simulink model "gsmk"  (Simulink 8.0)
settings: Solver=ode45  SolverMode=SingleTasking  StartTime=0.0  StopTime=3.0  RelTol=1e-3  AbsTol=1e-6
undefined symbols (not defined in the file or in its folder): DiscIntNeverNeededParam

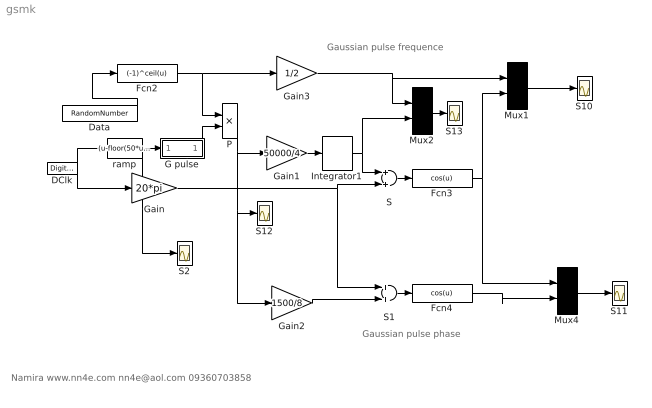
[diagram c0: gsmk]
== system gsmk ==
  note: Gaussian pulse phase
  note: Gaussian pulse frequence
  note: Namira www.nn4e.com nn4e@aol.com 09360703858
  DClk : DigitalClock  SampleTime=0.0005
  Data : RandomNumber  Variance=10  Seed=100  SampleTime=1*pi/50
  Fcn2 : Fcn  Expr=(-1)^ceil(u)
  Fcn3 : Fcn  Expr=cos(u)
  Fcn4 : Fcn  Expr=cos(u)
  G pulse : Subsystem
  Gain : Gain  Gain=20*pi
  Gain1 : Gain  Gain=50000/4
  Gain2 : Gain  Gain=1500/8
  Gain3 : Gain  Gain=1/2
  Integrator1 : DiscreteIntegrator  SampleTime=0.0001  UpperSaturationLimit=1  LowerSaturationLimit=-1  ICPrevOutput=DiscIntNeverNeededParam  ICPrevScaledInput=DiscIntNeverNeededParam
  Mux1 : Mux  Inputs=2
  Mux2 : Mux  Inputs=2
  Mux4 : Mux  Inputs=2
  P : Product
  S : Sum
  S1 : Sum
  S{2,10..13} (5 alike) : Scope
  ramp : Fcn  Expr=(u-floor(50*u/pi)*pi/50)*50/pi-1/2
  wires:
  ramp/1 -> G pulse/1(In1), S2/1
  G pulse/1(Out1) -> P/2
  Gain1/1 -> Integrator1/1
  P/1 -> Gain1/1, S12/1, Gain2/1
  Fcn2/1 -> P/1, Gain3/1
  Mux1/1 -> S10/1
  S/1 -> Fcn3/1
  Fcn3/1 -> Mux1/2, Mux4/1
  DClk/1 -> Gain/1, ramp/1
  Gain/1 -> S/2, S1/1
  S1/1 -> Fcn4/1
  Gain2/1 -> S1/2
  Data/1 -> Fcn2/1
  Integrator1/1 -> S/1, Mux2/2
  Mux2/1 -> S13/1
  Gain3/1 -> Mux1/1, Mux2/1
  Mux4/1 -> S11/1
  Fcn4/1 -> Mux4/2

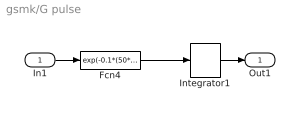
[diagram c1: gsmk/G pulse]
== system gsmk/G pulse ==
  In1 : Inport
  Fcn4 : Fcn  Expr=exp(-0.1*(50*u/pi+1/2)*(50*u/pi+1/2))-exp(-0.1*(50*u/pi-1/2)*(50*u/pi-1/2))
  Integrator1 : DiscreteIntegrator  SampleTime=0.0001  UpperSaturationLimit=1  LowerSaturationLimit=-1  ICPrevOutput=DiscIntNeverNeededParam  ICPrevScaledInput=DiscIntNeverNeededParam
  Out1 : Outport  InitialOutput=0
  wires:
  In1/1 -> Fcn4/1
  Integrator1/1 -> Out1/1
  Fcn4/1 -> Integrator1/1
